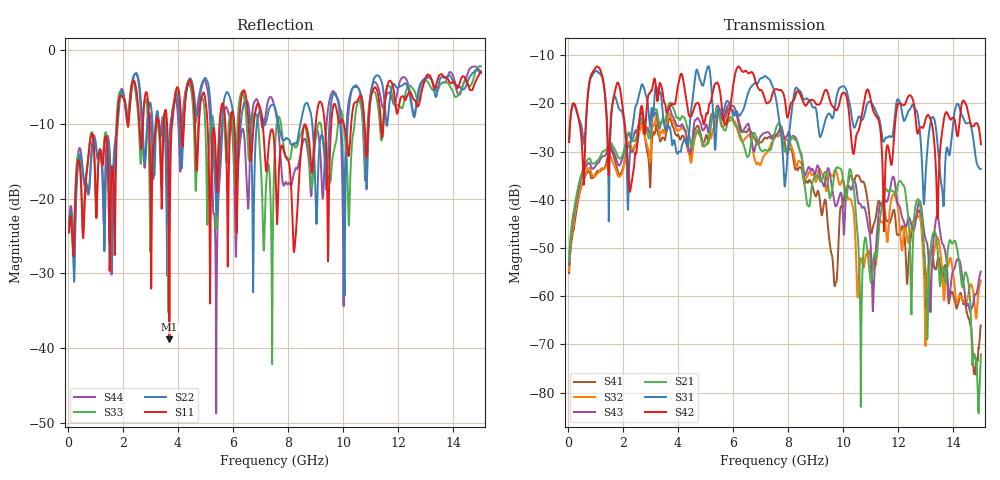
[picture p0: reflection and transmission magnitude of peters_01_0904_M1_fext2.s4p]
# MHZ S RI R 50.00
! FREQ  S11  S12  S13  S14
!  S21  S22  S23  S24
!  S31  S32  S33  S34
!  S41  S42  S43  S44
!  REAL  IMAG  REAL  IMAG  REAL  IMAG  REAL  IMAG
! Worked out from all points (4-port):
!   1496 points, 50 MHz to 15 GHz, reference 50 ohm
!   strongest paths, dB at 50 MHz, 3.79 GHz, 7.53 GHz, 11.27 GHz, 15 GHz:
!     S42: -28.0, -20.0, -17.1, -23.2, -28.5
!     S31: -28.0, -28.6, -18.3, -22.7, -33.6
!     S21: -52.8, -20.6, -25.8, -48.2, -72.1
!     S43: -53.4, -22.5, -26.7, -43.9, -54.9
!     S32: -54.7, -23.5, -27.1, -45.9, -56.8
!     S41: -55.3, -24.5, -26.6, -40.5, -66.1
!   lowest |S11| = -38.9 dB at 3.69 GHz (marker M1), VSWR 1.02, Z = 51.1 - j0.288 ohm
!   |S11| at or under -10 dB: start of sweep to 1.792 GHz; 5.074 GHz to 5.519 GHz (444.4 MHz wide, 8.39 % of centre); 7.079 GHz to 8.607 GHz (1.528 GHz wide, 19.5 % of centre)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
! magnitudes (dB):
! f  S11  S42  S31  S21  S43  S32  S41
! 50 MHz  -24.5  -28.0  -28.0  -52.8  -53.4  -54.7  -55.3
! 3.69 GHz  -38.9  -20.6  -24.8  -20.0  -20.9  -22.1  -23.1
! 9.72 GHz  -7.4  -21.3  -19.9  -33.8  -41.3  -33.9  -57.5
! 10.27 GHz  -11.0  -25.7  -21.2  -33.8  -37.8  -40.0  -35.0
! 10.65 GHz  -6.2  -23.3  -23.2  -73.2  -41.2  -52.1  -36.2
! 12.1 GHz  -6.4  -20.1  -20.7  -36.3  -42.6  -49.0  -46.2
! 15 GHz  -3.0  -28.5  -33.6  -72.1  -54.9  -56.8  -66.1
